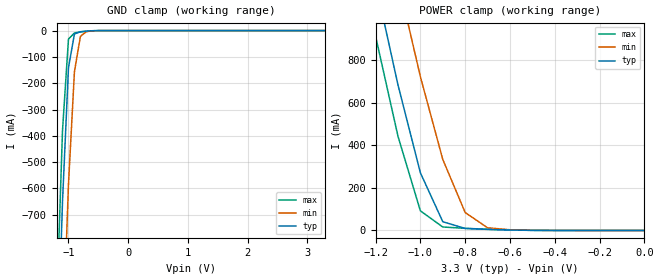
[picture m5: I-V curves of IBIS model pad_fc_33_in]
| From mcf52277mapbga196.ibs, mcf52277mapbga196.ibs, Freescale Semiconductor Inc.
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|   Model Pad_fc_in
[Model]   pad_fc_33_in
Model_type   Input
Polarity   Non-Inverting
Vinl =   0.9900V
Vinh =   2.3100V
C_comp   8.5000pF   8.5000pF   8.5000pF
[Temperature Range]   25.0000   0.1500k   -40.0000
[Voltage Range]   3.3000V   3.0000V   3.6000V
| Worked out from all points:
|   GND clamp passes 1 mA (typ) near -0.63 V on its own axis
|   POWER clamp passes 1 mA (typ) near -0.52 V on its own axis
[GND_clamp]
| voltage   I(typ)   I(min)   I(max)
-3.3V     -18.48A    -18.65A    -18.42A
-1.2V     -1.357A    -1.942A    -1.067A
-1.1V     -650.5mA   -1.219A    -380mA
-1V       -141.2mA   -584.4mA   -32.29mA
-900mV    -12.85mA   -155.8mA   -8.89mA
-800mV    -4.42mA    -21.92mA   -5.229mA
-700mV    -2.049mA   -3.904mA   -2.397mA
-400mV    -7.776uA   -47.99uA   -2.574uA
3.3V      2.182uA    34.68uA    1.661uA
[POWER_clamp]
| voltage   I(typ)   I(min)   I(max)
-3.3V     12.25A     12.55A     12.11A
-1.3V     1.667A     2.163A     1.421A
-1.2V     1.163A     1.662A     913.9mA
-1.1V     684.8mA    1.177A     443.1mA
-1V       271.3mA    723.4mA    92.34mA
-900mV    41.22mA    334.1mA    16.32mA
-800mV    9.5mA      84.35mA    10.09mA
-700mV    5.131mA    12.62mA    5.713mA
-600mV    2.291mA    3.316mA    2.385mA
-500mV    581uA      1.097mA    477.4uA
0V        2.182uA    2.618uA    2.249uA
